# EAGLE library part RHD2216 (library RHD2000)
Intan Technologies RHD2216 chip
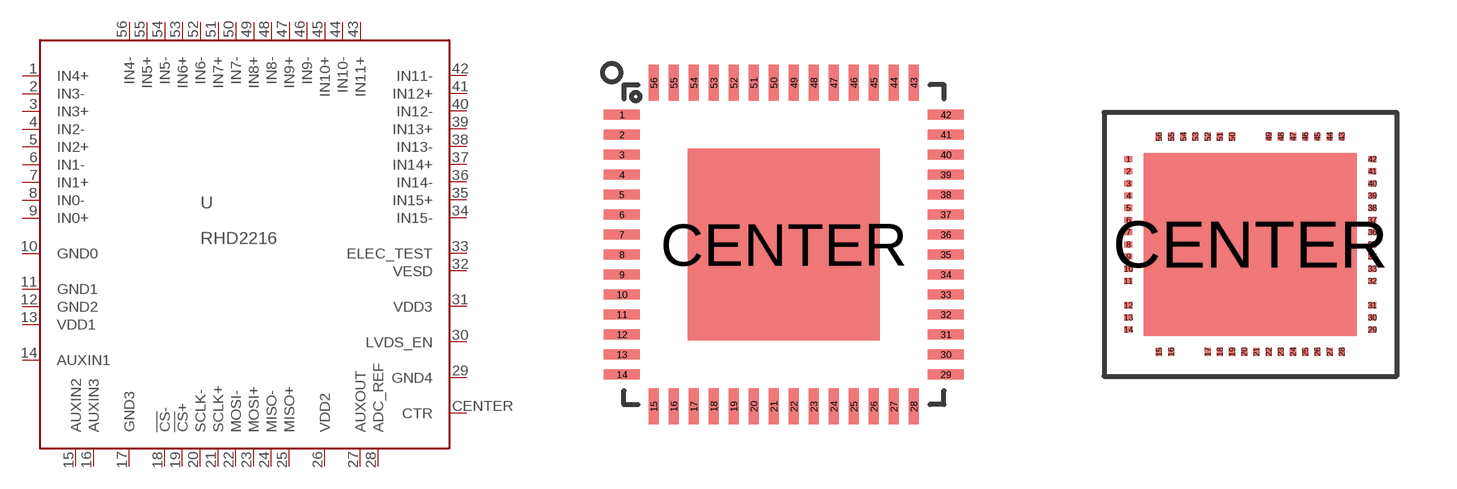
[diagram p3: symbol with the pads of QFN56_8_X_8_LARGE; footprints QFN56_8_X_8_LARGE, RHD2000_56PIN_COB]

Designator prefix U

## RHD2216_QFN  [QFN56_8_X_8_LARGE]
1  IN4+  in
2  IN3-  in
3  IN3+  in
4  IN2-  in
5  IN2+  in
6  IN1-  in
7  IN1+  in
8  IN0-  in
9  IN0+  in
10  GND0  in
11  GND1  pwr
12  GND2  pwr
13  VDD1  pwr
14  AUXIN1  in
15  AUXIN2  in
16  AUXIN3  in
17  GND3  pwr
18  !CS!-  in
19  !CS!+  in
20  SCLK-  in
21  SCLK+  in
22  MOSI-  in
23  MOSI+  in
24  MISO-  out
25  MISO+  out
26  VDD2  pwr
27  AUXOUT  hiz
28  ADC_REF  pas
29  GND4  pwr
30  LVDS_EN  in
31  VDD3  pwr
32  VESD  pwr
33  ELEC_TEST  in
34  IN15-  in
35  IN15+  in
36  IN14-  in
37  IN14+  in
38  IN13-  in
39  IN13+  in
40  IN12-  in
41  IN12+  in
42  IN11-  in
43  IN11+  in
44  IN10-  in
45  IN10+  in
46  IN9-  in
47  IN9+  in
48  IN8-  in
49  IN8+  in
50  IN7-  in
51  IN7+  in
52  IN6-  in
53  IN6+  in
54  IN5-  in
55  IN5+  in
56  IN4-  in
CENTER  CTR  pwr

## RHD2216_COB  [RHD2000_56PIN_COB]
Pads as for QFN56_8_X_8_LARGE

## Footprint QFN56_8_X_8_LARGE (pad centres in mm)
smd 0.9 x 0.25: 1 -4.05,3.25; 2 -4.05,2.75; 3 -4.05,2.25; 4 -4.05,1.75; 5 -4.05,1.25; 6 -4.05,0.75; 7 -4.05,0.25; 8 -4.05,-0.25; 9 -4.05,-0.75; 10 -4.05,-1.25; 11 -4.05,-1.75; 12 -4.05,-2.25; 13 -4.05,-2.75; 14 -4.05,-3.25; 29 4.05,-3.25; 30 4.05,-2.75; 31 4.05,-2.25; 32 4.05,-1.75; 33 4.05,-1.25; 34 4.05,-0.75; 35 4.05,-0.25; 36 4.05,0.25; 37 4.05,0.75; 38 4.05,1.25; 39 4.05,1.75; 40 4.05,2.25; 41 4.05,2.75; 42 4.05,3.25
smd 0.25 x 0.9: 15 -3.25,-4.05; 16 -2.75,-4.05; 17 -2.25,-4.05; 18 -1.75,-4.05; 19 -1.25,-4.05; 20 -0.75,-4.05; 21 -0.25,-4.05; 22 0.25,-4.05; 23 0.75,-4.05; 24 1.25,-4.05; 25 1.75,-4.05; 26 2.25,-4.05; 27 2.75,-4.05; 28 3.25,-4.05; 43 3.25,4.05; 44 2.75,4.05; 45 2.25,4.05; 46 1.75,4.05; 47 1.25,4.05; 48 0.75,4.05; 49 0.25,4.05; 50 -0.25,4.05; 51 -0.75,4.05; 52 -1.25,4.05; 53 -1.75,4.05; 54 -2.25,4.05; 55 -2.75,4.05; 56 -3.25,4.05
smd 4.8 x 4.8: CENTER 0,0

## Footprint RHD2000_56PIN_COB (pad centres in mm)
smd 0.203 x 0.152: 1 -3.048,2.134; 2 -3.048,1.829; 3 -3.048,1.524; 4 -3.048,1.219; 5 -3.048,0.914; 6 -3.048,0.61; 7 -3.048,0.305; 8 -3.048,0; 9 -3.048,-0.305; 10 -3.048,-0.61; 11 -3.048,-0.914; 12 -3.048,-1.524; 13 -3.048,-1.829; 14 -3.048,-2.134; 29 3.048,-2.134; 30 3.048,-1.829; 31 3.048,-1.524; 32 3.048,-0.914; 33 3.048,-0.61; 34 3.048,-0.305; 35 3.048,0; 36 3.048,0.305; 37 3.048,0.61; 38 3.048,0.914; 39 3.048,1.219; 40 3.048,1.524; 41 3.048,1.829; 42 3.048,2.134
smd 0.152 x 0.203: 15 -2.286,-2.692; 16 -1.981,-2.692; 17 -1.067,-2.692; 18 -0.762,-2.692; 19 -0.457,-2.692; 20 -0.152,-2.692; 21 0.152,-2.692; 22 0.457,-2.692; 23 0.762,-2.692; 24 1.067,-2.692; 25 1.372,-2.692; 26 1.676,-2.692; 27 1.981,-2.692; 28 2.286,-2.692; 43 2.286,2.692; 44 1.981,2.692; 45 1.676,2.692; 46 1.372,2.692; 47 1.067,2.692; 48 0.762,2.692; 49 0.457,2.692; 50 -0.457,2.692; 51 -0.762,2.692; 52 -1.067,2.692; 53 -1.372,2.692; 54 -1.676,2.692; 55 -1.981,2.692; 56 -2.286,2.692
smd 5.334 x 4.572: CENTER 0,0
